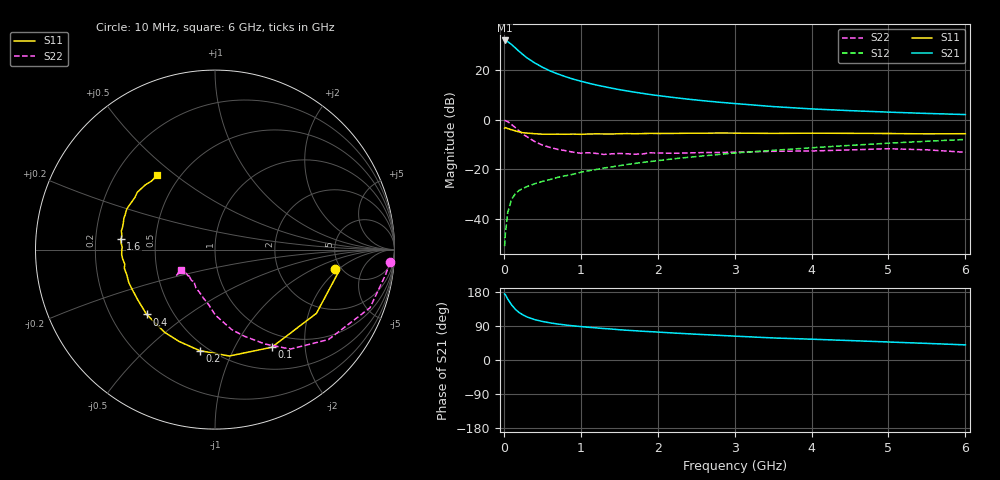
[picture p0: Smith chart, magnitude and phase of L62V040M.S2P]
!  INFINEON TECHNOLOGIES Small Signal Semiconductors
! BFR380L3 , Si-NPN RF-Transistor in TSLP-3-1
!  Vce=2 V,  Ic=40 mA
! Common Emitter S-Parameters:  07. March 2005
#  GHz  S  MA  R  50
! f  S11  S21  S12  S22
! GHz  Mag  Ang  Mag  Ang  Mag  Ang  Mag  Ang
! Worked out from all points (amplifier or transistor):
!   36 points, 10 MHz to 6 GHz, reference 50 ohm
!   highest |S21| = 32.1 dB at 10 MHz (marker M1)
!   |S21| within 3 dB of that: start of sweep to 149.1 MHz
!   unconditionally stable (mu >= 1): 1.632 GHz to 4.876 GHz
!   at 250 MHz: K = 0.45, MSG = 27.0 dB, |S12| = -27.7 dB
!   at 1.4 GHz: K = 0.98, MSG = 15.9 dB, |S12| = -19.0 dB
!   at 6 GHz: K = 0.98, MSG = 5.0 dB, |S12| = -7.9 dB
!   S11 on the Smith chart (normalised r, x): 10 MHz: 4.47, -1.74; 100 MHz: 0.79, -1.43; 200 MHz: 0.45, -0.75; 400 MHz: 0.36, -0.35; 1.6 GHz: 0.31, +0.05; 6 GHz: 0.38, +0.43
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0.01  0.6762 -9.0  40.2 174.4  0.0028 77.6  0.9788 -4.0
0.02  0.6982 -10.6  39.85 172.4  0.005 87.5  0.9604 -8.4
0.05  0.6675 -32.1  38.12 161.1  0.0133 78.3  0.9223 -20.6
0.1  0.6296 -59.8  33.28 145.6  0.0247 66.7  0.8068 -38.4
0.15  0.5982 -82.3  28.38 133.6  0.0322 58.6  0.6958 -52.8
0.2  0.5692 -98.6  24.08 125.0  0.0376 55.9  0.5954 -62.1
0.25  0.5495 -111.4  20.73 118.8  0.0412 53.3  0.5094 -71.3
0.3  0.5395 -121.3  17.97 113.7  0.0447 52.7  0.4562 -78.1
0.4  0.5249 -136.5  14.18 106.6  0.0511 52.6  0.3649 -89.7
0.5  0.5136 -146.4  11.62 101.8  0.0568 54.3  0.3091 -96.5
0.6  0.5118 -153.6  9.767 98.0  0.062 55.5  0.2775 -103.5
0.7  0.5143 -158.8  8.473 95.0  0.0687 57.3  0.2526 -110.2
0.9  0.5157 -168.5  6.655 90.2  0.0795 59.5  0.2218 -120.9
1.1  0.5172 -174.3  5.508 86.4  0.0934 61.6  0.2165 -126.7
1.3  0.5192 -179.9  4.704 83.0  0.1062 62.9  0.2001 -134.4
1.6  0.5284 173.6  3.839 78.5  0.1249 63.7  0.2063 -141.3
2.2  0.5312 164.2  2.836 71.3  0.1627 64.6  0.2109 -143.6
2.8  0.5411 155.4  2.271 65.0  0.2 64.7  0.2184 -149.1
3.5  0.5324 147.1  1.853 58.2  0.2418 62.6  0.2313 -147.9
4.5  0.5337 140.8  1.534 51.3  0.3049 60.8  0.2466 -147.0
5.5  0.5204 132.8  1.347 43.8  0.3694 56.9  0.2477 -146.8
6  0.5246 127.8  1.279 39.9  0.4015 54.7  0.2211 -149.8
